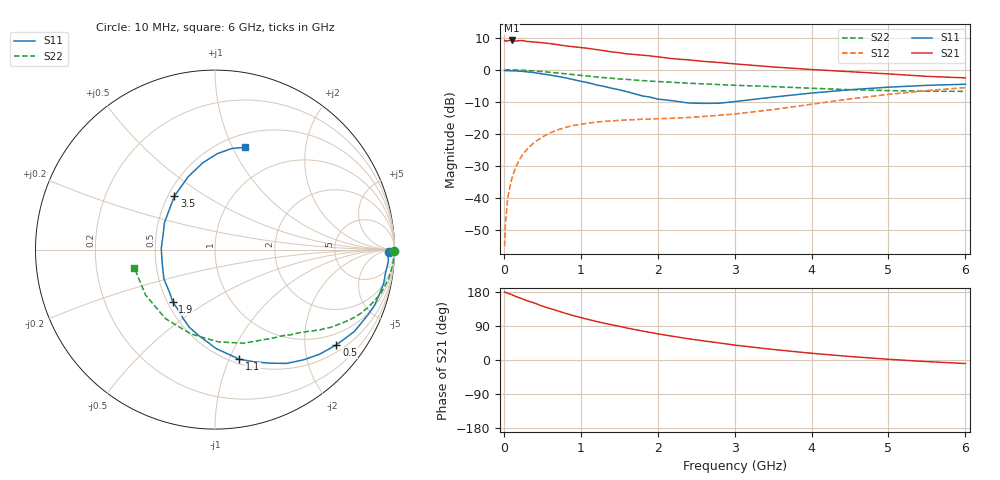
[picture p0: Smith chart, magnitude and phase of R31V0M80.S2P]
! SIEMENS Small Signal Semiconductors
! BFR181
! Si NPN RF Bipolar Junction Transistor in SOT23
! VCE = 1 V  IC = 0.8 mA
! Common Emitter S-Parameters:  May  1996
# GHz  S  MA  R  50
!  f  S11  S21  S12  S22
! GHz  MAG  ANG  MAG  ANG  MAG  ANG  MAG  ANG
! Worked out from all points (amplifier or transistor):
!   36 points, 10 MHz to 6 GHz, reference 50 ohm
!   highest |S21| = 9.1 dB at 100 MHz (marker M1)
!   |S21| within 3 dB of that: start of sweep to 1.25 GHz
!   unconditionally stable (mu >= 1): 2.057 GHz to 4.016 GHz
!   at 250 MHz: K = 0.15, MSG = 17.6 dB, |S12| = -26.2 dB
!   at 1.4 GHz: K = 0.74, MSG = 10.7 dB, |S12| = -15.9 dB
!   at 6 GHz: K = 0.93, MSG = 1.5 dB, |S12| = -5.6 dB
!   S11 on the Smith chart (normalised r, x): 10 MHz: 51, -21; 500 MHz: 0.68, -2.75; 1.1 GHz: 0.54, -1.09; 1.9 GHz: 0.53, -0.36; 3.5 GHz: 0.54, +0.38; 6 GHz: 0.64, +1.12
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0.01  0.9673 -0.8  2.844 179.6  0.0018 80.0  0.9983 -0.3
0.02  0.9629 -1.5  2.779 178.5  0.0038 87.6  0.993 -0.7
0.05  0.9684 -3.8  2.821 176.3  0.0101 87.3  0.9963 -1.9
0.1  0.9588 -7.7  2.849 172.7  0.0196 84.0  0.9955 -3.8
0.15  0.9583 -11.4  2.793 168.1  0.0296 81.6  0.991 -5.7
0.25  0.9414 -19.4  2.831 160.6  0.0488 76.9  0.9809 -9.3
0.4  0.9004 -30.5  2.694 150.2  0.0749 70.1  0.957 -14.5
0.5  0.8598 -38.1  2.627 142.1  0.0897 65.4  0.9335 -17.8
0.6  0.8242 -45.0  2.548 135.9  0.104 61.2  0.9105 -20.8
0.8  0.7486 -57.9  2.349 123.3  0.1264 53.8  0.8641 -25.9
1  0.6609 -71.0  2.212 112.0  0.1417 48.3  0.8153 -30.3
1.1  0.6255 -77.5  2.144 106.9  0.1479 45.9  0.7929 -32.3
1.4  0.5152 -94.9  1.893 92.9  0.1595 40.3  0.7356 -37.5
1.6  0.4554 -108.4  1.762 84.4  0.1656 38.3  0.7064 -40.0
1.9  0.3744 -129.0  1.641 72.8  0.1701 37.5  0.664 -44.0
2.2  0.3282 -150.1  1.482 62.5  0.176 37.6  0.6363 -48.2
2.4  0.3033 -166.2  1.421 56.0  0.1804 39.2  0.6152 -51.0
2.8  0.3008 164.0  1.293 45.0  0.1956 42.0  0.5869 -57.5
3.5  0.3747 127.1  1.103 27.8  0.2399 45.7  0.5458 -72.8
4.5  0.4881 98.1  0.93 9.2  0.3504 43.1  0.4888 -105.9
5.5  0.5708 80.6  0.788 -4.3  0.4733 31.0  0.4623 -146.8
6  0.5939 73.7  0.746 -9.2  0.5266 23.1  0.4609 -167.4
